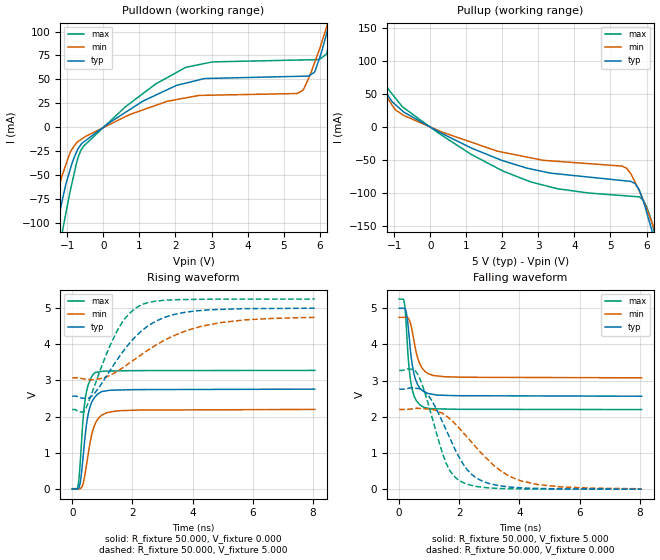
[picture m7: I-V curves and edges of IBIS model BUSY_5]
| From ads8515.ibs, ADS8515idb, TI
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|   BUSY OUTPUT Model  5V
[Model] BUSY_5
Model_type Output
Polarity   Non-Inverting
Enable   Active-Low
Vmeas = 2.5
Vref = 2.5
Cref = 15pF
Rref = 50
|   typ   min   max
| AVERAGE
C_comp   5.4569220E-12   4.7181840E-12   6.4344025E-12
| HIGH state
|C_comp   5.5875520E-12   4.9215320E-12   6.4582620E-12
| LOW state
|C_comp   5.3262920E-12   4.5148360E-12   6.4105430E-12
[Voltage Range]   5   4.75   5.25
[Temperature Range]   27   85   -40
[Pullup Reference]   5   4.75   5.25
[Pulldown Reference]   0   0   0
[Power Clamp Reference]   5   4.75   5.25
[GND Clamp Reference]   0   0   0
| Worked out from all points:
|   slope of the pulldown table from 0 to 0.75 V, typ, clamps not added: 39.8 ohm
|   slope of the pullup table from 0 to 0.75 V, typ, clamps not added: 35.1 ohm
|   falling waveform, R_fixture 50.000, V_fixture 5.000: 20-80 % time 239ps typ, 297ps min, 194ps max; typ from 5 V to 2.57 V
|   rising waveform, R_fixture 50.000, V_fixture 0.000: 20-80 % time 249ps typ, 311ps min, 199ps max; typ from 0 V to 2.76 V
|   rising waveform, R_fixture 50.000, V_fixture 5.000: 20-80 % time 1.44ns typ, 2.15ns min, 967ps max; typ from 2.57 V to 5 V
|   falling waveform, R_fixture 50.000, V_fixture 0.000: 20-80 % time 1.01ns typ, 1.57ns min, 726ps max; typ from 2.76 V to 0 V
[Pulldown]
|   Voltage   I  typ   I  min   I  max
-5V       -984.7mA   -723.4mA   -1.34A
-1.761V   -208.4mA   -139.7mA   -297.9mA
-1.37V    -122.2mA   -80.94mA   -174mA
-1.119V   -72.91mA   -47.86mA   -105.4mA
-744mV    -25.94mA   -16.34mA   -37.32mA
-545.9mV  -15.49mA   -11.05mA   -19.73mA
2.301V    46.2mA     30.73mA    62.73mA
5.377V    53.14mA    35.17mA    70.17mA
5.852V    57.34mA    66.66mA    70.56mA
6.196V    98.25mA    105.3mA    77.48mA
6.619V    160.3mA    156mA      148.9mA
9.985V    693mA      585.6mA    836.7mA
[Pullup]
|   Voltage   I  typ   I  min   I  max
-5V       615.3mA    503.4mA    781.6mA
-2.908V   300mA      247.6mA    374mA
-1.765V   128.2mA    108mA      154.4mA
-1.148V   46.08mA    40.95mA    56.65mA
-732.2mV  22.72mA    17.68mA    29.26mA
224.2mV   -6.719mA   -5.085mA   -8.905mA
2.785V    -63.51mA   -46.59mA   -83.21mA
5.327V    -81.13mA   -59.26mA   -104mA
5.786V    -94.08mA   -95.52mA   -105.9mA
6.143V    -156.4mA   -143.6mA   -143.4mA
6.23V     -174.7mA   -156.9mA   -162.7mA
9.985V    -1.074A    -835.6mA   -1.369A
[Ramp]
R_load = 50
|   typ   min   max
dV/dt_r   1.65662/2.47591e-010   1.34624/3.07109e-010   1.96736/1.98317e-010
dV/dt_f   1.48099/2.37347e-010   1.01943/2.92385e-010   1.83103/1.93018e-010
[Falling Waveform]
R_fixture = 50.000
V_fixture = 5.000
V_fixture_min = 4.750
V_fixture_max = 5.250
C_fixture = 0.000
|  time   V  typ   V  min   V  max
0s        4.997V     4.744V     5.25V
135ps     4.995V     4.745V     5.247V
178.4ps   4.995V     4.745V     5.118V
236.8ps   4.882V     4.745V     4.505V
321.5ps   4.312V     4.7V       3.425V
431.1ps   3.462V     4.375V     2.764V
624.7ps   2.872V     3.596V     2.39V
803.1ps   2.703V     3.304V     2.267V
1.506ns   2.592V     3.105V     2.214V
8.06ns    2.567V     3.075V     2.198V
[Rising Waveform]
R_fixture = 50.000
V_fixture = 0.000
V_fixture_min = 0.000
V_fixture_max = 0.000
C_fixture = 0.000
|  time   V  typ   V  min   V  max
0s        619.2nV    10.79mV    578.2nV
204.7ps   18.94mV    9.763mV    160.5mV
279.7ps   259.8mV    20.78mV    934.6mV
367.9ps   956.8mV    176.4mV    2.025V
468.5ps   1.76V      644.3mV    2.678V
586.7ps   2.264V     1.255V     2.997V
769.7ps   2.558V     1.816V     3.222V
994ps     2.696V     2.051V     3.252V
1.506ns   2.736V     2.163V     3.265V
8.06ns    2.761V     2.201V     3.279V
[Rising Waveform]
R_fixture = 50.000
V_fixture = 5.000
V_fixture_min = 4.750
V_fixture_max = 5.250
C_fixture = 0.000
|  time   V  typ   V  min   V  max
0s        2.567V     3.075V     2.198V
396.6ps   2.508V     3.041V     2.151V
763.3ps   2.67V      3.027V     2.907V
1.495ns   3.576V     3.254V     4.378V
1.874ns   3.999V     3.468V     4.832V
2.284ns   4.357V     3.705V     5.087V
3.116ns   4.758V     4.135V     5.218V
4.345ns   4.939V     4.507V     5.244V
5.751ns   4.985V     4.675V     5.248V
8.06ns    4.997V     4.744V     5.25V
[Falling Waveform]
R_fixture = 50.000
V_fixture = 0.000
V_fixture_min = 0.000
V_fixture_max = 0.000
C_fixture = 0.000
|  time   V  typ   V  min   V  max
0s        2.761V     2.201V     3.279V
621.1ps   2.78V      2.234V     3.173V
1.07ns    2.466V     2.205V     2.051V
1.555ns   1.649V     2.027V     731.7mV
1.788ns   1.224V     1.861V     392.2mV
2.113ns   712mV      1.575V     186.8mV
2.775ns   218mV      958mV      53.23mV
3.36ns    90.97mV    516.7mV    17.38mV
4.038ns   37.21mV    232.8mV    8.203mV
8.06ns    619.2nV    10.79mV    578.2nV
